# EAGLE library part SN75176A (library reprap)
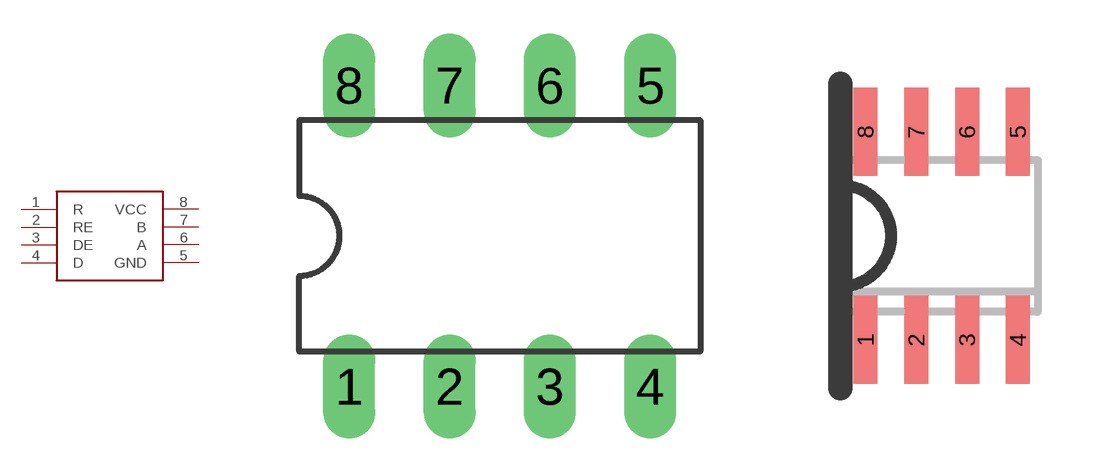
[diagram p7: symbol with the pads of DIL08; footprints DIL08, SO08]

Designator prefix -

## SN75176ADIL  [DIL08]
1  R
2  RE
3  DE
4  D
5  GND
6  A
7  B
8  VCC

## SN75176ASOIC  [SO08]
Pads as for DIL08

## Footprint DIL08 (pad centres in mm)
Dual In Line Package
drill 0.813 long: 1 -3.81,-3.81; 2 -1.27,-3.81; 3 1.27,-3.81; 4 3.81,-3.81; 5 3.81,3.81; 6 1.27,3.81; 7 -1.27,3.81; 8 -3.81,3.81

## Footprint SO08 (pad centres in mm)
SMALL OUTLINE INTEGRATED CIRCUIT body 3.9 mm/JEDEC MS-012AA
smd 0.6 x 2.2: 1 -1.905,-2.6; 2 -0.635,-2.6; 3 0.635,-2.6; 4 1.905,-2.6; 5 1.905,2.6; 6 0.635,2.6; 7 -0.635,2.6; 8 -1.905,2.6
